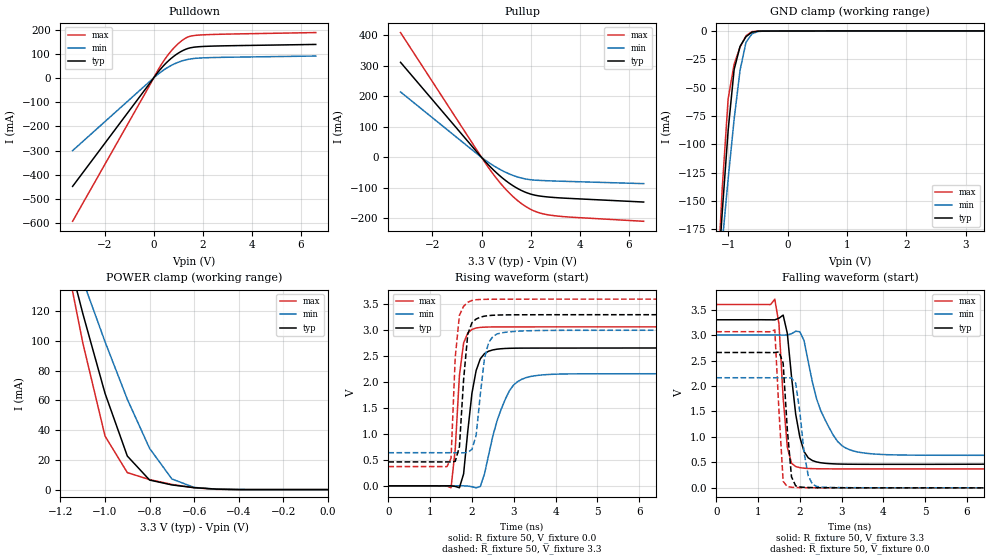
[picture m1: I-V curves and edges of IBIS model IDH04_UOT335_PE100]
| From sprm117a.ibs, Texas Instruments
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[Model]   IDH04_UOT335_PE100
| I/O with pulldown
Model_type   I/O
Vinh = 2.00
Vinl = 0.80
Enable   Active-Low
Polarity   Non-Inverting
| signals   A, GZ, Y
Vmeas = 1.5
|   typ   min   max
C_comp   3.033p   2.954p   3.045p
|   typ   min   max
[Temperature Range]   25   -40   125
|   typ   min   max
[Voltage Range]   3.30V   3.00V   3.60V
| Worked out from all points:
|   slope of the pulldown table from 0 to 0.495 V, typ, clamps not added: 8.22 ohm
|   slope of the pullup table from 0 to 0.495 V, typ, clamps not added: 11.8 ohm
|   GND clamp passes 1 mA (typ) near -0.60 V on its own axis
|   POWER clamp passes 1 mA (typ) near -0.57 V on its own axis
|   rising waveform, R_fixture 50, V_fixture 0.0: 20-80 % time 241ps typ, 478ps min, 164ps max; typ from 0 V to 2.66 V
|   falling waveform, R_fixture 50, V_fixture 3.3: 20-80 % time 257ps typ, 560ps min, 159ps max; typ from 3.3 V to 0.462 V
|   rising waveform, R_fixture 50, V_fixture 3.3: 20-80 % time 157ps typ, 205ps min, 134ps max; typ from 0.462 V to 3.3 V
|   falling waveform, R_fixture 50, V_fixture 0.0: 20-80 % time 141ps typ, 200ps min, 124ps max; typ from 2.66 V to 0 V
[Pulldown]
|   Voltage   I(typ)   I(min)   I(max)
-3.3V     -448.2mA   -300.5mA   -592.5mA
200mV     26.69mA    17.06mA    36.54mA
600mV     70.53mA    44.94mA    97.01mA
800mV     87.84mA    55.83mA    121.2mA
1.1V      108.3mA    68.43mA    150.3mA
1.4V      121.9mA    76.68mA    169.3mA
1.9V      129.3mA    82.24mA    177.4mA
6.6V      138.4mA    90.43mA    187.4mA
[GND_clamp]
|   Voltage   I(typ)   I(min)   I(max)
-3.3V     -2.116A    -1.593A    -2.736A
-1.2V     -239.6mA   -245.7mA   -241.4mA
-1.1V     -160mA     -186.9mA   -138.9mA
-1V       -87.4mA    -130.4mA   -59.63mA
-900mV    -34.08mA   -77.98mA   -29.34mA
-800mV    -13.51mA   -34.6mA    -14.21mA
-700mV    -4.989mA   -9.98mA    -4.207mA
-600mV    -1.01mA    -2.466mA   -549.8uA
-500mV    -132.7uA   -459.7uA   -91.89uA
-400mV    -40.94uA   -74.05uA   -56.3uA
3.3V      100.8uA    56.39uA    177.3uA
[Pullup]
|   Voltage   I(typ)   I(min)   I(max)
-3.3V     311.6mA    214.5mA    409mA
-200mV    18.62mA    12.57mA    24.84mA
300mV     -26.32mA   -17.35mA   -35.69mA
900mV     -70.83mA   -45.77mA   -97.06mA
1.2V      -88.69mA   -56.59mA   -122.3mA
1.5V      -103.4mA   -64.99mA   -143.8mA
1.8V      -114.7mA   -70.84mA   -161.1mA
2.1V      -122.5mA   -74.08mA   -174.1mA
2.7V      -129.7mA   -76.64mA   -188.1mA
3.6V      -134.5mA   -78.95mA   -195.7mA
6.6V      -146.3mA   -86mA      -209.4mA
[POWER_clamp]
|   Voltage   I(typ)   I(min)   I(max)
-3.3V     1.526A     1.156A     1.976A
-1.2V     176.8mA    183.8mA    174.5mA
-1.1V     118.5mA    140.8mA    98.81mA
-1V       64.71mA    99.4mA     35.99mA
-900mV    22.55mA    60.73mA    11.42mA
-800mV    6.422mA    27.7mA     6.719mA
-700mV    3.145mA    7.155mA    3.485mA
-600mV    1.32mA     1.456mA    1.225mA
-500mV    313.2uA    317.8uA    181.3uA
-400mV    30.64uA    44.8uA     9.582uA
0V        1pA        1pA        1pA
[Ramp]
|   I(typ)   I(min)   I(max)
dV/dt_r   1.594/0.232n   1.297/0.473n   1.839/0.145n
dV/dt_f   1.703/0.252n   1.417/0.556n   1.937/0.152n
[Rising Waveform]
R_fixture = 50
V_fixture = 0.0
|  pu_on
|  TIME   V(typ)   V(min)   V(max)
0s        2nV        12nV       1nV
1.5ns     547.5uV    45.48uV    -36.07mV
1.6ns     -10.77mV   234.5uV    704.5mV
1.7ns     -36.67mV   487.8uV    2.126V
1.8ns     229.6mV    581.7uV    2.754V
2ns       1.787V     -16.42mV   3.016V
2.3ns     2.549V     230.8mV    3.06V
2.8ns     2.649V     1.675V     3.064V
3.3ns     2.656V     2.088V     3.065V
10ns      2.657V     2.162V     3.066V
[Falling Waveform]
R_fixture = 50
V_fixture = 3.3
V_fixture_min = 3.0
V_fixture_max = 3.6
|  pd_on
|  TIME   V(typ)   V(min)   V(max)
0s        3.3V       3V         3.6V
1.4ns     3.298V     3V         3.705V
1.5ns     3.331V     2.999V     3.215V
1.6ns     3.392V     2.999V     1.768V
1.7ns     3.033V     3.001V     799.3mV
1.9ns     1.447V     3.075V     418.9mV
2.2ns     589.7mV    2.477V     380.5mV
2.6ns     483mV      1.342V     373.6mV
3.2ns     464.1mV    745.6mV    372.3mV
10ns      461.6mV    639mV      372mV
[Rising Waveform]
R_fixture = 50
V_fixture = 3.3
V_fixture_min = 3.0
V_fixture_max = 3.6
|  pd_off
|  TIME   V(typ)   V(min)   V(max)
0s        461.6mV    638.9mV    372mV
1.4ns     461.7mV    638.9mV    369.9mV
1.5ns     460.9mV    639.2mV    532.4mV
1.6ns     472.2mV    639.1mV    2.48V
1.7ns     753.4mV    638.2mV    3.288V
1.9ns     2.924V     643.7mV    3.539V
2ns       3.145V     703.2mV    3.575V
2.3ns     3.272V     2.461V     3.596V
2.6ns     3.292V     2.928V     3.598V
10ns      3.3V       3V         3.6V
[Falling Waveform]
R_fixture = 50
V_fixture = 0.0
|  pu_off
|  TIME   V(typ)   V(min)   V(max)
0s        2.657V     2.162V     3.066V
1.4ns     2.656V     2.162V     3.102V
1.6ns     2.448V     2.161V     129.1mV
1.7ns     1.144V     2.163V     23.59mV
1.8ns     215.6mV    2.156V     11.45mV
1.9ns     38.63mV    2.054V     7.173mV
2.1ns     10.62mV    694.4mV    3.064mV
2.2ns     7.584mV    239.2mV    2.25mV
2.4ns     4.137mV    28.41mV    1.289mV
10ns      256nV      6.691uV    12.63uV
